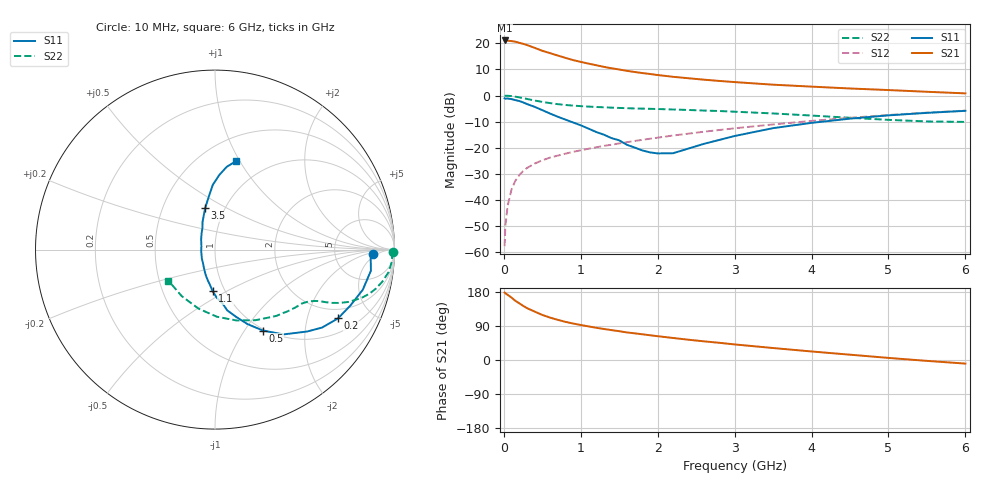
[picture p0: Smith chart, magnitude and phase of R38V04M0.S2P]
! SIEMENS Small Signal Semiconductors
! BFR181
! Si NPN RF Bipolar Junction Transistor in SOT23
! VCE = 8 V  IC = 4 mA
! Common Emitter S-Parameters:  May  1996
# GHz  S  MA  R  50
!  f  S11  S21  S12  S22
! GHz  MAG  ANG  MAG  ANG  MAG  ANG  MAG  ANG
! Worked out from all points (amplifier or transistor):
!   36 points, 10 MHz to 6 GHz, reference 50 ohm
!   highest |S21| = 21.1 dB at 10 MHz (marker M1)
!   |S21| within 3 dB of that: start of sweep to 415.2 MHz
!   unconditionally stable (mu >= 1): 1.311 GHz to 3.168 GHz
!   at 250 MHz: K = 0.35, MSG = 24.4 dB, |S12| = -28.9 dB
!   at 1.4 GHz: K = 1.02, MAG = 13.8 dB, |S12| = -18.9 dB
!   at 6 GHz: K = 0.86, MSG = 3.3 dB, |S12| = -5.8 dB
!   S11 on the Smith chart (normalised r, x): 10 MHz: 15, -3; 200 MHz: 1.56, -3.12; 500 MHz: 0.98, -1.22; 1.1 GHz: 0.88, -0.43; 3.5 GHz: 0.81, +0.40; 6 GHz: 0.73, +0.97
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0.01  0.8805 -1.6  11.34 177.9  0.0013 82.1  0.9938 -0.8
0.02  0.8687 -3.0  11.33 176.2  0.0032 89.4  0.9874 -1.5
0.05  0.8766 -7.7  11.24 171.9  0.0078 84.9  0.988 -3.8
0.1  0.8532 -15.2  11.02 164.6  0.0159 81.8  0.9753 -7.4
0.15  0.8155 -22.6  10.73 156.2  0.0233 77.1  0.9489 -10.9
0.2  0.7852 -29.2  10.23 149.7  0.0297 74.2  0.9216 -13.7
0.25  0.7385 -36.0  9.784 143.0  0.0357 70.7  0.8929 -16.1
0.3  0.6873 -41.6  9.281 137.0  0.0408 69.1  0.86 -18.2
0.4  0.6071 -51.1  8.189 127.8  0.0496 65.9  0.8018 -21.3
0.5  0.5239 -59.4  7.188 118.9  0.0574 63.5  0.7544 -23.2
0.6  0.452 -66.5  6.485 112.0  0.0647 62.2  0.7161 -24.5
0.7  0.3925 -72.6  5.84 106.0  0.0705 61.8  0.683 -25.4
0.8  0.3455 -78.6  5.261 100.7  0.0769 61.2  0.6587 -26.0
0.9  0.3047 -81.9  4.771 96.3  0.0833 61.2  0.6401 -26.6
1.1  0.2323 -93.3  4.088 88.7  0.0955 61.4  0.6135 -27.9
1.3  0.1778 -102.8  3.542 81.9  0.1085 61.7  0.5937 -29.2
1.6  0.1137 -123.9  2.971 72.8  0.1277 61.9  0.5715 -31.6
2.2  0.0784 165.2  2.282 58.1  0.1714 60.9  0.5396 -38.3
3.5  0.2371 103.4  1.612 31.6  0.2791 53.3  0.4533 -60.2
4.5  0.3604 92.0  1.363 14.0  0.3743 43.7  0.3743 -88.3
5.5  0.4652 82.0  1.179 -2.3  0.4699 31.6  0.3188 -125.6
6  0.5086 76.4  1.099 -9.5  0.5138 24.9  0.3121 -146.5
